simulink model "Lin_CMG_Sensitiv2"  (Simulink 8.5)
settings: Solver=ode3  StartTime=0.0  StopTime=3000  FixedStep=Ts  RelTol=1e-3
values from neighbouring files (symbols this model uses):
  Ave = [    [vehicle_flex34.m]    (also in vehicle_rigid.m)
  Bve = [    [vehicle_flex34.m]    (also in vehicle_rigid.m)
  Cve = [    [vehicle_flex34.m]    (also in vehicle_rigid.m)
  Dve = [    [vehicle_flex34.m]    (also in vehicle_rigid.m)
  J = [0.119416e9, -0.476e7,   -0.1216e7;     -0.476e7,     0.40408e8, -0.30121e6;     -0.1216e7,   -0.30121e6,  0.110166e9]    [start.m]    (also in start1.m; start2.m; start3.m)
  omg = 20*wo    (= 0.022)    [start.m]    (also in start1.m; start2.m; start3.m)
  r2d = 180/pi    (= 57.2957795131)    [start.m]    (also in start1.m; start2.m; start3.m)
  zeb = 0.95    [start.m]    (also in start1.m; start2.m; start3.m)
undefined symbols (not defined in the file or in its folder): Torq_Lim

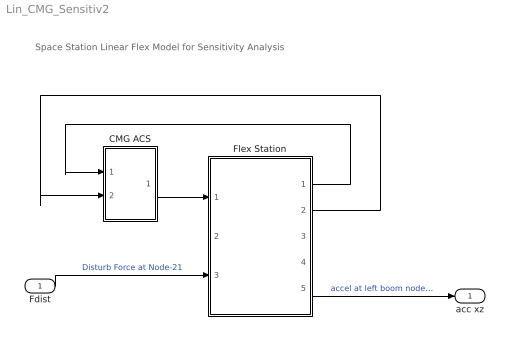
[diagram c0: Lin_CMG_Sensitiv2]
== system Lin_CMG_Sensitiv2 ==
  note: Space Station Linear Flex Model for Sensitivity Analysis
  Fdist : Inport
  CMG ACS : Subsystem
  Flex Station : Subsystem
  acc xz : Outport
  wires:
  Flex Station/1(wbf) -> CMG ACS/1(wb)
  Flex Station/2(att) -> CMG ACS/2(ater)
  CMG ACS/1(Tq) -> Flex Station/1(Tcmg)
  Fdist/1 -> Flex Station/3(Fdist)  "Disturb Force at Node-21"
  Flex Station/5(acc xz LB18) -> acc xz/1  "accel at left boom node 18"

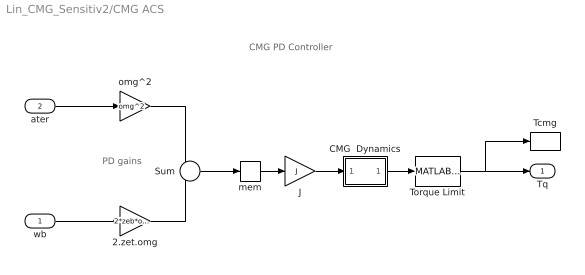
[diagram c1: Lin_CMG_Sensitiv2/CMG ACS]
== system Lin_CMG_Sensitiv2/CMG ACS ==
  note: CMG PD Controller
  note: PD gains
  wb : Inport
  ater : Inport  Port=2  PortDimensions=3
  2.zet.omg : Gain  Gain=2*zeb*omg
  CMG  Dynamics : Subsystem
  J : Gain  Gain=J  Multiplication=Matrix(K*u)
  Sum : Sum  Inputs=--
  Tcmg : ToWorkspace  VariableName=Tcmg  SampleTime=-1
  Torque Limit : MATLABFcn  MATLABFcn=Torq_Lim( u(1:3) )  OutputDimensions=3
  mem : Memory
  omg^2 : Gain  Gain=omg^2
  Tq : Outport
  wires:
  wb/1 -> 2.zet.omg/1
  Sum/1 -> mem/1
  2.zet.omg/1 -> Sum/2
  ater/1 -> omg^2/1
  omg^2/1 -> Sum/1
  J/1 -> CMG  Dynamics/1(I)
  mem/1 -> J/1
  CMG  Dynamics/1(O) -> Torque Limit/1
  Torque Limit/1 -> Tq/1, Tcmg/1

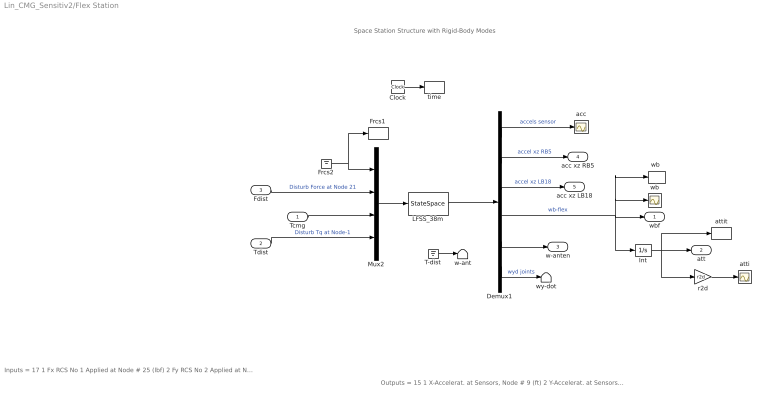
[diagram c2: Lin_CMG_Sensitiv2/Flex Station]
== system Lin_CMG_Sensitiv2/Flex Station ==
  note: Outputs = 15 1 X-Accelerat. at Sensors, Node # 9 (ft) 2 Y-Accelerat. at Sensors, Node # 9 (ft) 3 Z-Accelerat. at Sensors, Node # 9 (ft) 4 X-Accelerat. at Right Boom End, Node # 5 (ft) 5 Z-Accelerat. at Right Boom End, Node # 5 (ft) 6 X-Accelerat. at Left Boom End, Node # 18 (ft) 7 Z-Accelerat. at Left Boom End, Node # 18 (ft) 8 X-Rot. Rate at Sensors, Node # 9 (radian) 9 Y-Rot. Rate at Sensors, Node # 9 (radian) 10 Z-Rot. Rate at Sensors, Node # 9 (radian) 11 X-Rot. Rate at Antena Bot-Left, Node # 24 (radian) 12 Y-Rot. Rate at Antena Bot-Left, Node # 24 (radian) 13 Z-Rot. Rate at Antena Bot-Left, Node # 24 (radian) 14 Y-Rot.Accel. at Right Joint, Node # 7 (radian) 15 Y-Rot.Accel. at Left Joint, Node # 16 (radian)
  note: Inputs = 17 1 Fx RCS No 1 Applied at Node # 25 (lbf) 2 Fy RCS No 2 Applied at Node # 25 (lbf) 3 Fx RCS No 3 Applied at Node # 26 (lbf) 4 Fy RCS No 4 Applied at Node # 26 (lbf) 5 Fx RCS No 5 Applied at Node # 27 (lbf) 6 Fy RCS No 6 Applied at Node # 27 (lbf) 7 Fx RCS No 7 Applied at Node # 28 (lbf) 8 Fy RCS No 8 Applied at Node # 28 (lbf) 9 Fx Disturb. No 9 at Node # 21 (lbf) 10 Fy Disturb. No 10 at Node # 21 (lbf) 11 Fz Disturb. No 11 at Node # 21 (lbf) 12 Torq-x No 1 CMG Applied at Node # 10 (ft-lb) 13 Torq-y No 2 CMG Applied at Node # 10 (ft-lb) 14 Torq-z No 3 CMG Applied at Node # 10 (ft-lb) 15 Torq-x No 4 Gimbal Dist. at Node # 1 (ft-lb) 16 Torq-y No 5 Gimbal Dist. at Node # 1 (ft-lb) 17 Torq-z No 6 Gimbal Dist. at Node # 1 (ft-lb)
  note: Space Station Structure with Rigid-Body Modes
  Tcmg : Inport
  Tdist : Inport  Port=2
  Fdist : Inport  Port=3
  Clock : Clock
  Demux1 : Demux  Outputs=[3, 2, 2, 3, 3, 2]
  Frcs1 : ToWorkspace  VariableName=Frcs  SampleTime=-1
  Frcs2 : Ground
  Int : Integrator
  LFSS_38m : StateSpace  A=Ave  B=Bve  C=Cve  D=Dve  X0=0
  Mux2 : Mux  Inputs=[8, 3, 3, 3]
  T-dist : Ground
  acc : Scope
  atti : Scope
  attit : ToWorkspace  VariableName=atti  SampleTime=-1
  r2d : Gain  Gain=r2d
  time : ToWorkspace  VariableName=time  SampleTime=-1
  w-ant : Terminator
  wb : Scope
  "wb " : ToWorkspace  VariableName=wb  SampleTime=-1
  wy-dot : Terminator
  wbf : Outport
  att : Outport  Port=2
  w-anten : Outport  Port=3
  acc xz RB5 : Outport  Port=4
  acc xz LB18 : Outport  Port=5
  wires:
  Demux1/6 -> wy-dot/1  "wyd joints"
  Fdist/1 -> Mux2/2  "Disturb Force at Node 21"
  Demux1/3 -> acc xz LB18/1  "accel xz LB18"
  Demux1/2 -> acc xz RB5/1  "accel xz RB5"
  Tcmg/1 -> Mux2/3
  Demux1/4 -> wbf/1, Int/1, wb/1, "wb "/1  "wb-flex"
  Demux1/1 -> acc/1  "accels sensor"
  LFSS_38m/1 -> Demux1/1
  Clock/1 -> time/1
  Mux2/1 -> LFSS_38m/1
  r2d/1 -> atti/1
  Int/1 -> att/1, attit/1, r2d/1
  Frcs2/1 -> Mux2/1, Frcs1/1
  Tdist/1 -> Mux2/4  "Disturb Tq at Node-1"
  T-dist/1 -> w-ant/1
  Demux1/5 -> w-anten/1

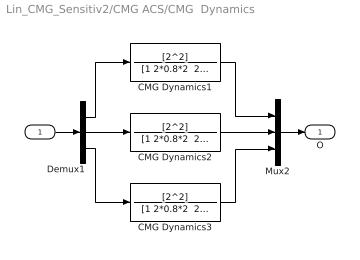
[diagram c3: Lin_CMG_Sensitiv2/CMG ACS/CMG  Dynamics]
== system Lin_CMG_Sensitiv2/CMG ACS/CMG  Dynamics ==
  I : Inport
  CMG Dynamics1 : TransferFcn  Numerator=[2^2]  Denominator="[1 2*0.8*2  2^2]"
  CMG Dynamics2 : TransferFcn  Numerator=[2^2]  Denominator="[1 2*0.8*2  2^2]"
  CMG Dynamics3 : TransferFcn  Numerator=[2^2]  Denominator="[1 2*0.8*2  2^2]"
  Demux1 : Demux  Outputs=3
  Mux2 : Mux  Inputs=3
  O : Outport
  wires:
  CMG Dynamics2/1 -> Mux2/2
  CMG Dynamics3/1 -> Mux2/3
  CMG Dynamics1/1 -> Mux2/1
  Demux1/2 -> CMG Dynamics2/1
  Demux1/1 -> CMG Dynamics1/1
  Demux1/3 -> CMG Dynamics3/1
  I/1 -> Demux1/1
  Mux2/1 -> O/1
